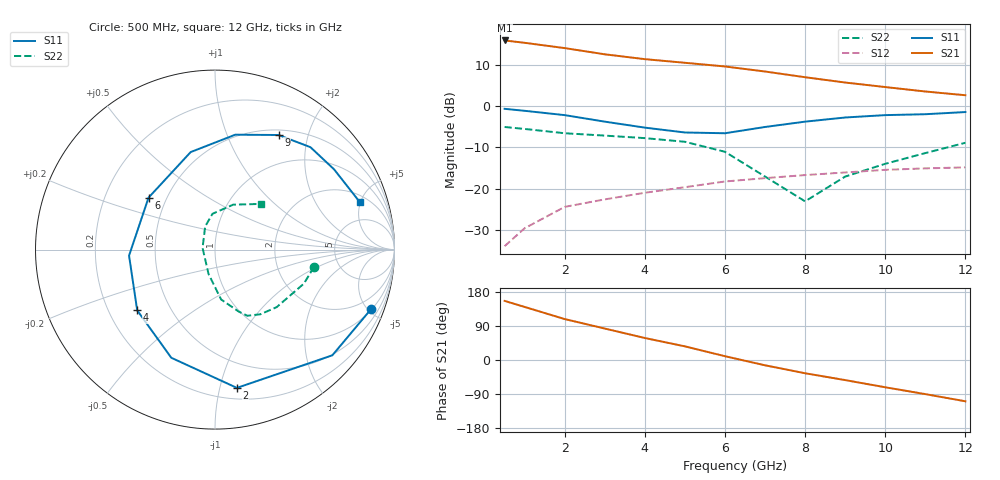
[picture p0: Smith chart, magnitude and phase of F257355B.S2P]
!ATF-257335
!S-PARAMETERS at Vds=5V  Id=50mA.  LAST UPDATED 07-22-92
# ghz s ma r 50
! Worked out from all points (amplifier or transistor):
!   13 points, 500 MHz to 12 GHz, reference 50 ohm
!   highest |S21| = 16.0 dB at 500 MHz (marker M1)
!   |S21| within 3 dB of that: start of sweep to 2.758 GHz
!   unconditionally stable (mu >= 1): 4.576 GHz to 8.161 GHz
!   at 2 GHz: K = 0.58, MSG = 19.3 dB, |S12| = -24.4 dB
!   at 6 GHz: K = 1.06, MAG = 12.5 dB, |S12| = -18.3 dB
!   at 12 GHz: K = 0.78, MSG = 8.8 dB, |S12| = -14.8 dB
!   S11 on the Smith chart (normalised r, x): 500 MHz: 1.05, -5.19; 2 GHz: 0.29, -1.13; 4 GHz: 0.32, -0.31; 6 GHz: 0.40, +0.30; 9 GHz: 0.57, +1.55; 12 GHz: 2.63, +4.97
0.5  0.93 -21.0  6.29 156.0  0.02 69.0  0.56 -10.0
1  0.88 -42.0  5.89 140.0  0.033 62.0  0.53 -21.0
2  0.78 -81.0  5.08 108.0  0.06 49.0  0.47 -43.0
3  0.65 -112.0  4.27 83.0  0.074 39.0  0.44 -55.0
4  0.55 -142.0  3.73 58.0  0.089 28.0  0.41 -64.0
5  0.48 -176.0  3.37 36.0  0.104 20.0  0.37 -69.0
6  0.47 142.0  3.04 10.0  0.122 6.0  0.28 -83.0
7  0.56 104.0  2.64 -14.0  0.134 -6.0  0.14 -105.0
8  0.65 80.0  2.25 -35.0  0.146 -17.0  0.07 172.0
9  0.73 61.0  1.94 -53.0  0.157 -26.0  0.14 113.0
10  0.78 47.0  1.71 -72.0  0.169 -40.0  0.2 94.0
11  0.8 34.0  1.51 -90.0  0.176 -53.0  0.27 68.0
12  0.85 18.0  1.36 -109.0  0.181 -64.0  0.36 45.0
